(* Logix 5000 AddOnInstructionDefinition export AMCI_NXFE2_Set_State; software revision 20.03 *)

ADD_ON_INSTRUCTION AMCI_NXFE2_Set_State   (* revision 1.0, vendor AMCI, ExecuteEnableInFalse *)
VAR_INPUT
   axis_status_bits : INT; {required}
   No_Fault_Output_0_OFF_1_ON : BOOL; {required}
   On_Line_Output_0_OFF_1_ON : BOOL; {required}
   Move_Complete_Output_0_OFF_1_ON : BOOL; {required}
END_VAR
VAR_IN_OUT
   NXFE2_output_data : _000A:NXFE2_0986AEB4:O:0; {required}
END_VAR
VAR_OUTPUT
   EN : BOOL; {access Read Only, visible}
   ER : BOOL; {access Read Only, visible}
END_VAR
VAR
   command_data_block : INT[10];
        [0]   // Command Bits MSW
        [1]   // Command Bits LSW
        [1].5   // set state bit
        [2]   // Upper Target Position
        [3]   // Lower Target Position
        [4]   // Upper Programmed Speed
        [5]   // Lower Programmed Speed
END_VAR

ROUTINE EnableInFalse   (* ladder *)
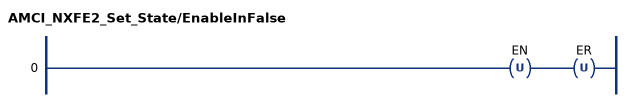
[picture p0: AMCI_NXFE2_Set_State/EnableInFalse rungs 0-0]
   0: OTU(EN)OTU(ER);
END_ROUTINE

ROUTINE Logic   (* ladder *)
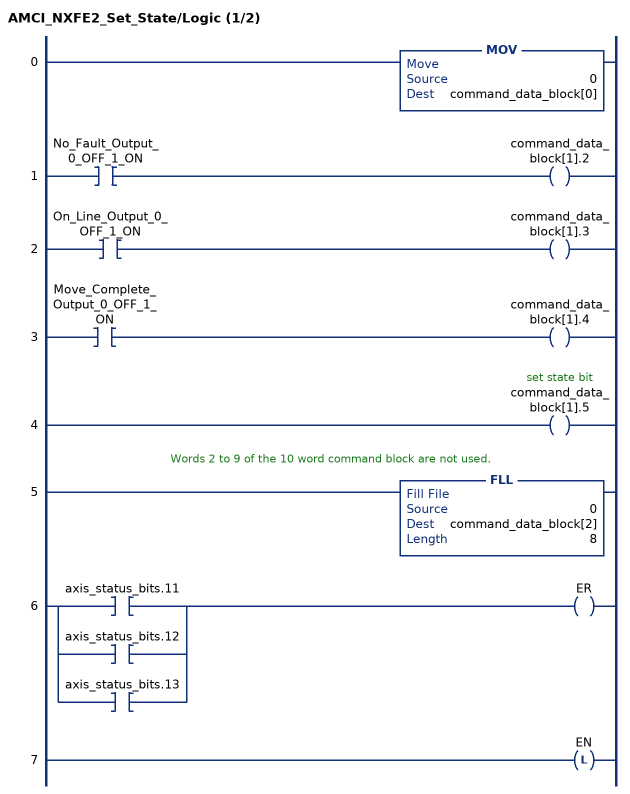
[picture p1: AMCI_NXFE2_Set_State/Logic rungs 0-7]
   0: MOV(0,command_data_block[0]);
   1: XIC(No_Fault_Output_0_OFF_1_ON)OTE(command_data_block[1].2);
   2: XIC(On_Line_Output_0_OFF_1_ON)OTE(command_data_block[1].3);
   3: XIC(Move_Complete_Output_0_OFF_1_ON)OTE(command_data_block[1].4);
   4: OTE(command_data_block[1].5);
   // Words 2 to 9 of the 10 word command block are not used.
   5: FLL(0,command_data_block[2],8);
   6: [XIC(axis_status_bits.11) ,XIC(axis_status_bits.12) ,XIC(axis_status_bits.13) ]OTE(ER);
   7: OTL(EN);
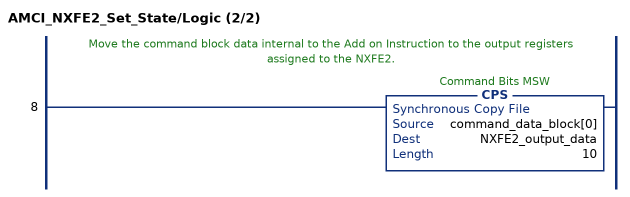
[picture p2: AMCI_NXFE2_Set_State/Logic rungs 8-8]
   // Move the command block data internal to the Add on Instruction to the output registers assigned to the NXFE2.
   8: CPS(command_data_block[0],NXFE2_output_data,10);
END_ROUTINE
END_ADD_ON_INSTRUCTION
